FUNCTION_BLOCK Example26_serialnumbers //at least 2 flyways (physical) - GetFlywaySerialNum, PMC_GetPMCSerialNum
VAR_INPUT
	Execute : BOOL;
END_VAR
VAR_OUTPUT
	Done : BOOL;
END_VAR
VAR_IN_OUT
	PM_Controller : PMControllerType;	// the planar motor controller to use
END_VAR
VAR
	PMC_GetPMCVersion1 : PMC_GetPMCVersion;
	PMC_GetPMCSerialNum1 : PMC_GetPMCSerialNum;
	PMC_GetFlywaySerialNum1 : PMC_GetFlywaySerialNum;
	PMC_GetFlywaySerialNum2 : PMC_GetFlywaySerialNum;
END_VAR

//at least 2 flyways (physical) - GetFlywaySerialNum, PMC_GetPMCSerialNum, PMC_GetPMCVersion

//read software version number of the PMC
PMC_GetPMCVersion1(Execute := Execute,PM_Controller := PM_Controller);

//read serial number of the PMC
PMC_GetPMCSerialNum1(Execute := PMC_GetPMCVersion1.Done,PM_Controller := PM_Controller);

//read serial number of flyway 1
PMC_GetFlywaySerialNum1(Execute := PMC_GetPMCSerialNum1.Valid,FlywayID := 1,PM_Controller := PM_Controller);

//read serial number of flyway 2
PMC_GetFlywaySerialNum2(Execute := PMC_GetFlywaySerialNum1.Valid,FlywayID := 2,PM_Controller := PM_Controller);

Done := PMC_GetFlywaySerialNum2.Valid;

END_FUNCTION_BLOCK
